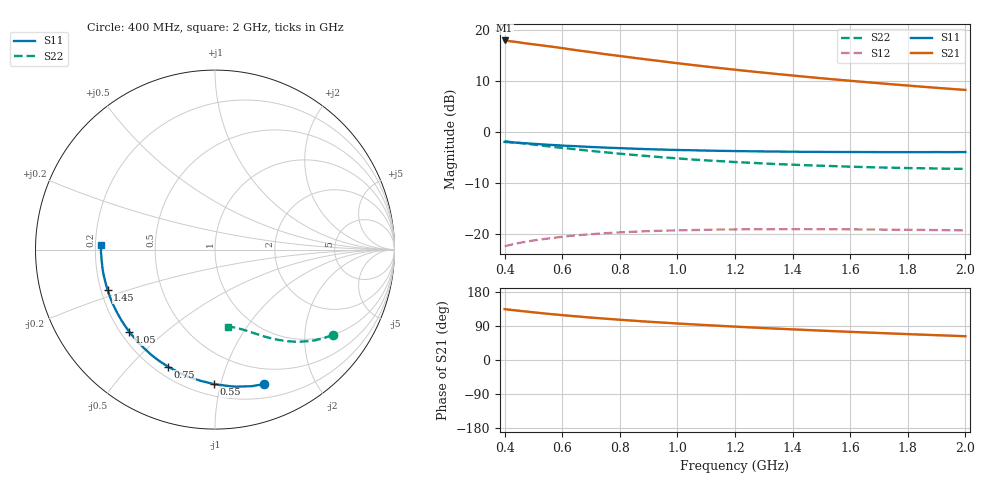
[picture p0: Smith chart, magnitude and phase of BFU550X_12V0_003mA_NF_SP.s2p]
! Filename:  P:\Prog\Test\Noise\ATS_data\Testdata_Net\BFU550X no attenuator noise\BFU550X_APG2013_44_C05_12p0V_003mA_NF_CM01_D.sf
! Date/Time: Fri 26/Jul/2013 14:37:14
! BFU550X_APG2013_44_C05_12p0V_1to10mA_NF_CM01_Bias3_R.sf
! Noise Parameter Data File
! BFU550X_APG2013_44_C05_12p0V_1to10mA_NF_CM01
! Date/time: Thu Jul 25 09:36:35 2013
! VAR V_out= 12.001000
! VAR I_out= 3.000000
! VAR V_in= 0.791800
! VAR I_in= 0.026505
! Device data file deembeded for feedlines and parallel
! Original file: \BFU550X no attenuator noise\BFU550X_APG2013_44_C05_12p0V_003mA_NF_CM01_R.sf
! Feed-files: PR005V01_100713_Feed1.s2p, PR005V01_100713_Feed2.s2p
! Parallel-file: PR005V01_100713_Par.s2p
# MHz S MA R 50
!  Freq-MHz  S11-mag  S11-arg  S21-mag  S21-arg  S12-mag  S12-arg  S22-mag  S22-arg
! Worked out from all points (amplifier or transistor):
!   37 points, 400 MHz to 2 GHz, reference 50 ohm
!   highest |S21| = 17.9 dB at 400 MHz (marker M1)
!   |S21| within 3 dB of that: start of sweep to 794.7 MHz
!   unconditionally stable (mu >= 1): nowhere
!   at 500 MHz: K = 0.19, MSG = 19.2 dB, |S12| = -21.2 dB
!   at 1.1 GHz: K = 0.40, MSG = 16.0 dB, |S12| = -19.1 dB
!   at 2 GHz: K = 0.74, MSG = 13.7 dB, |S12| = -19.2 dB
!   lowest NFmin = 0.60 dB at 460 MHz
!   S11 on the Smith chart (normalised r, x): 400 MHz: 0.33, -1.37; 550 MHz: 0.28, -0.95; 750 MHz: 0.25, -0.65; 1.05 GHz: 0.23, -0.38; 1.45 GHz: 0.23, -0.17; 2 GHz: 0.22, +0.02
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400  0.7984 -70.1  7.832 134.2  0.07648 51.8  0.8115 -36.1
420  0.7911 -72.9  7.691 132.4  0.07874 50.5  0.7968 -37.5
440  0.7854 -75.8  7.581 130.8  0.0811 49.2  0.7872 -38.5
480  0.7729 -81.2  7.295 127.5  0.08507 46.7  0.7622 -41.0
550  0.7497 -90.4  6.891 121.9  0.0908 42.6  0.7233 -44.9
600  0.7356 -96.2  6.594 118.4  0.09445 40.1  0.6982 -47.3
650  0.7248 -101.7  6.281 115.1  0.09767 37.8  0.6752 -49.4
700  0.7124 -107.0  6.022 111.9  0.1001 35.7  0.6519 -51.5
750  0.7029 -111.7  5.749 109.0  0.1024 33.9  0.6324 -53.3
800  0.694 -116.5  5.521 106.2  0.1042 32.1  0.6126 -55.1
850  0.6862 -120.9  5.292 103.6  0.106 30.4  0.5956 -56.6
900  0.6777 -125.1  5.083 101.0  0.1073 29.0  0.58 -58.1
950  0.6724 -129.0  4.884 98.6  0.1083 27.6  0.5641 -59.7
1050  0.6619 -136.2  4.519 94.2  0.1098 25.3  0.538 -62.3
1100  0.6572 -139.6  4.352 92.1  0.1105 24.2  0.5271 -63.4
1200  0.6502 -145.9  4.056 88.1  0.1115 22.3  0.508 -65.7
1350  0.643 -154.4  3.671 82.6  0.112 20.1  0.4845 -68.8
1450  0.6395 -159.5  3.45 79.2  0.1121 18.9  0.4724 -70.7
1500  0.6378 -161.9  3.346 77.5  0.1121 18.3  0.4671 -71.7
1600  0.6364 -166.6  3.161 74.3  0.1116 17.4  0.4576 -73.5
1750  0.6343 -172.9  2.914 69.8  0.1109 16.4  0.4466 -76.2
2000  0.6363 177.5  2.572 62.8  0.1091 15.7  0.435 -80.3
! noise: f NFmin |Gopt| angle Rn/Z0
400  0.6544  0.3325  29.92  0.1541
460  0.5973  0.323  42.27  0.1316
600  0.7241  0.3411  47.93  0.1497
800  0.7316  0.326  69.38  0.1256
1000  0.7952  0.3363  84.21  0.1153
1200  0.8263  0.3746  102.2  0.1005
1400  0.9142  0.3831  113.2  0.0963
1600  0.8691  0.3996  129.4  0.0761
1800  0.9221  0.437  142.7  0.0619
2000  0.9925  0.47  154.8  0.0509
